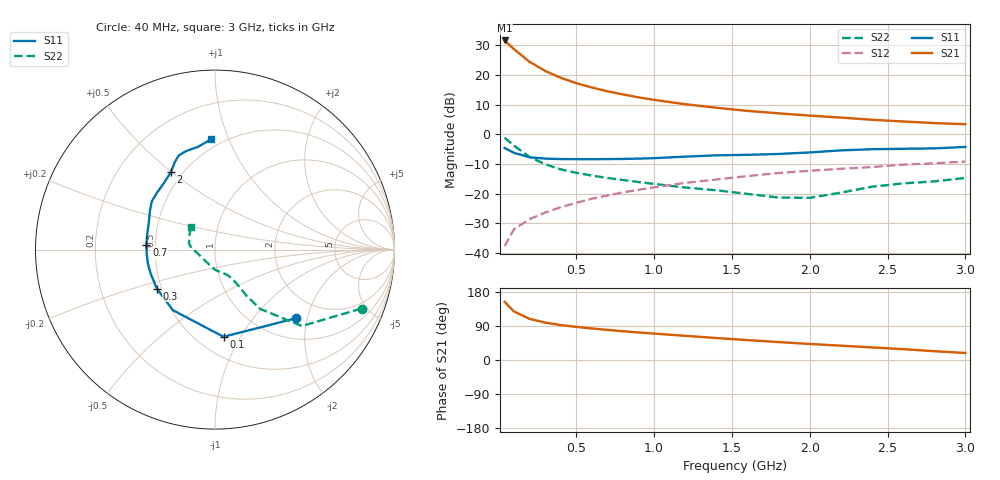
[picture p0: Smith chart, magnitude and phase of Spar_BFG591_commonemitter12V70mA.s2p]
! Filename:  BFG591G.S2P  Version:  4.0
! NXP part #: BFG591  Date: Jun 1994
! Bias condition: Vce=12V; Ic=70mA
#  MHz  S  MA  R  50
! Freq  S11  S21  S12  S22  !GUM [dB]
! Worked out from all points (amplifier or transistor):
!   21 points, 40 MHz to 3 GHz, reference 50 ohm
!   highest |S21| = 31.7 dB at 40 MHz (marker M1)
!   |S21| within 3 dB of that: start of sweep to 101.8 MHz
!   unconditionally stable (mu >= 1): 627.8 MHz to 2.179 GHz
!   at 300 MHz: K = 0.84, MSG = 23.9 dB, |S12| = -26.4 dB
!   at 1 GHz: K = 1.05, MAG = 13.4 dB, |S12| = -17.9 dB
!   at 3 GHz: K = 0.95, MSG = 6.3 dB, |S12| = -9.2 dB
!   S11 on the Smith chart (normalised r, x): 40 MHz: 1.45, -1.70; 100 MHz: 0.67, -0.85; 300 MHz: 0.47, -0.24; 700 MHz: 0.45, +0.03; 2 GHz: 0.43, +0.50; 3 GHz: 0.44, +0.86
40  0.59 -40.5  38.43 153.5  0.013 72.6  0.88 -21.9
100  0.488 -84.4  27.44 128.1  0.025 62.0  0.645 -41.3
200  0.411 -124.8  16.77 108.6  0.037 60.2  0.417 -52.6
300  0.39 -146.2  11.79 98.7  0.048 62.3  0.313 -55.7
400  0.383 -159.7  9.034 92.2  0.059 64.5  0.257 -56.6
500  0.382 -169.5  7.319 87.4  0.07 66.0  0.225 -57.6
600  0.381 -177.2  6.178 83.2  0.082 66.5  0.202 -58.6
700  0.383 176.2  5.341 79.4  0.093 67.0  0.184 -60.0
800  0.385 170.0  4.718 75.9  0.105 67.0  0.17 -61.8
900  0.39 163.9  4.217 72.6  0.116 67.0  0.157 -64.3
1000  0.397 158.4  3.822 69.7  0.128 66.6  0.146 -67.8
1200  0.421 149.5  3.229 63.8  0.152 65.2  0.127 -77.3
1400  0.443 142.6  2.814 58.0  0.173 63.4  0.114 -88.4
1600  0.452 135.9  2.492 52.5  0.198 62.2  0.099 -101.0
1800  0.467 127.7  2.264 47.3  0.223 59.1  0.086 -118.0
2000  0.496 119.8  2.074 42.3  0.243 57.3  0.085 -147.4
2200  0.537 114.6  1.92 37.8  0.263 55.1  0.104 -171.6
2400  0.562 111.1  1.764 33.2  0.281 54.1  0.131 176.7
2600  0.572 106.4  1.651 28.6  0.309 50.4  0.149 166.2
2800  0.58 99.6  1.55 23.2  0.325 46.5  0.161 152.7
3000  0.614 92.1  1.485 18.6  0.348 45.0  0.184 137.1
